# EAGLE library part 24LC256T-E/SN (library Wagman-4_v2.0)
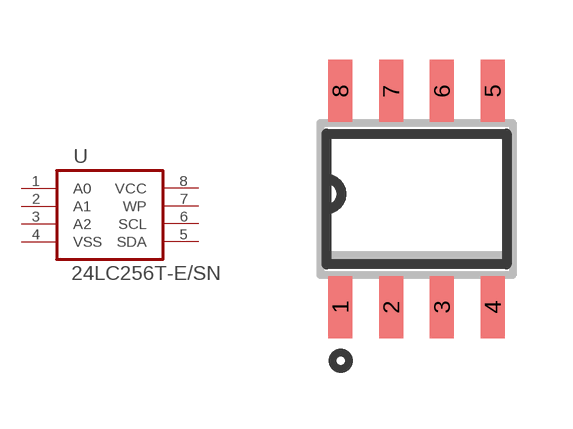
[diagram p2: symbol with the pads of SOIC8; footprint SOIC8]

Designator prefix U

## 24LC256T-E/SN  [SOIC8]
1  A0  pwr
2  A1  pas
3  A2  pas
4  VSS  pas
5  SDA  pas
6  SCL  pas
7  WP  pas
8  VCC  pas

## Footprint SOIC8 (pad centres in mm)
Small Outline IC
smd 0.6 x 1.55: 1 -1.905,-2.7; 2 -0.635,-2.7; 3 0.635,-2.7; 4 1.905,-2.7; 5 1.905,2.7; 6 0.635,2.7; 7 -0.635,2.7; 8 -1.905,2.7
